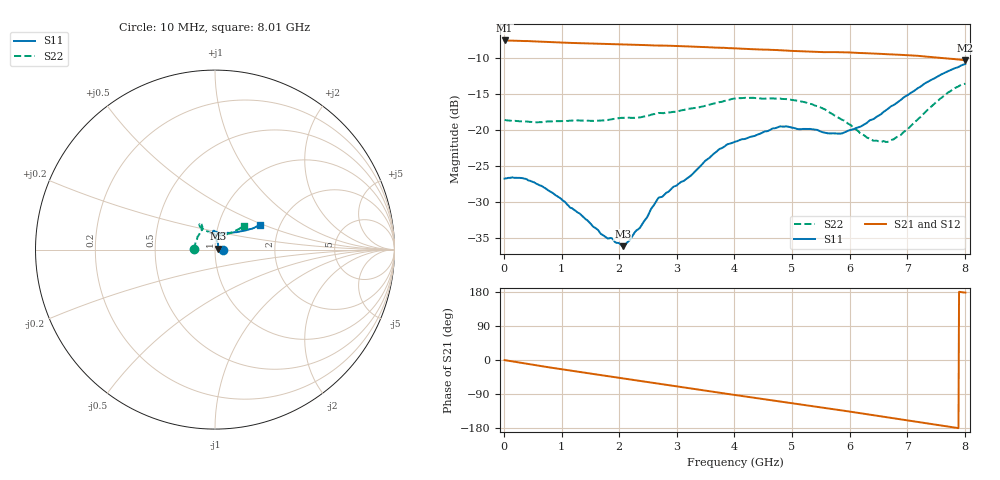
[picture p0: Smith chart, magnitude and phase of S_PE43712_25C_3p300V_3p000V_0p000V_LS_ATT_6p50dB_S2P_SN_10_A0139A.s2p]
! DEVICE ID: PE43712
! File Path: z:\PE43713\PE43713_CHAR_NOM_04292014\AMB\3p300\LS_ATT_6p50dB\PE43713_AMB_3p300V_3p000V_0p000V_LS_ATT_6p50dB_S2P_SN_10_A0139A.s2p
! Serial: 10
! Lot: A0139A
! Temp: 25C
! VDD: 3.300
! VSS: 0.000
! Control_Hi: 3.000
! Control_Lo: 0.000
! Attenuation Step: 6.50dB
! Port 1: RF1
! Port 2: RF2
! ThroughPath:1-2
! IDD: 0.0001471273
! ISS: -1.096e-007
#  Hz  S  RI  R  50
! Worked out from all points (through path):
!   801 points, 10 MHz to 8.01 GHz, reference 50 ohm
!   highest |S21| = -7.63 dB at 10 MHz (marker M1); lowest = -10.4 dB at 8.01 GHz (marker M2)
!   group delay of S21, straight-line fit = 62.5 ps
!   lowest |S11| = -36.1 dB at 2.06 GHz (marker M3), VSWR 1.03, Z = 51.5 + j0.513 ohm
!   |S11| at or under -10 dB: start of sweep to end of sweep
!   |S22| runs from -21.7 to -13.6 dB; largest |S21 - S12| = 0.0014
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1e7  0.0459 -6.25e-05  0.4156 -0.00229  0.4155 -0.00229  -0.1171 0.000707
3e8  0.0457 -0.00756  0.4088 -0.0557  0.4086 -0.0557  -0.1139 0.01
5.4e8  0.0413 -0.0114  0.3975 -0.0965  0.3976 -0.0966  -0.1113 0.0171
9.6e8  0.0314 -0.0127  0.3692 -0.1612  0.3693 -0.1612  -0.1103 0.0312
1.35e9  0.0234 -0.00989  0.3357 -0.2131  0.3357 -0.2131  -0.107 0.0439
1.71e9  0.0184 -0.00333  0.2993 -0.2557  0.2994 -0.2557  -0.1005 0.0578
2.06e9  0.0148 0.00498  0.2592 -0.2919  0.2592 -0.2918  -0.0969 0.0724
2.15e9  0.0152 0.00702  0.248 -0.3003  0.2481 -0.3002  -0.0948 0.0756
2.37e9  0.0152 0.0148  0.2195 -0.3189  0.2194 -0.3188  -0.0872 0.0854
2.68e9  0.0176 0.0287  0.1779 -0.3393  0.1779 -0.3393  -0.0777 0.1049
3.23e9  0.0104 0.0464  0.0984 -0.3641  0.0984 -0.3642  -0.0727 0.1195
3.72e9  0.00565 0.0722  0.0271 -0.3694  0.0268 -0.3694  -0.0732 0.1362
4.01e9  -0.000122 0.0826  -0.015 -0.3663  -0.015 -0.3662  -0.0802 0.1437
4.79e9  -0.00921 0.105  -0.1189 -0.3349  -0.1189 -0.3352  -0.0868 0.1397
5.35e9  0.00116 0.1007  -0.1822 -0.2959  -0.1821 -0.2957  -0.0825 0.1255
5.63e9  0.013 0.0935  -0.2103 -0.2737  -0.2102 -0.2738  -0.0674 0.1149
5.88e9  0.0265 0.091  -0.2363 -0.2504  -0.2358 -0.2505  -0.0497 0.1059
6.39e9  0.0714 0.0935  -0.2764 -0.1939  -0.2759 -0.1937  -0.0052 0.0847
6.68e9  0.1044 0.0954  -0.2935 -0.1577  -0.2932 -0.1577  0.0252 0.0791
6.99e9  0.1392 0.1011  -0.3072 -0.1174  -0.3067 -0.1174  0.0556 0.0825
7.71e9  0.2225 0.1239  -0.3107 -0.0224  -0.3105 -0.0227  0.1378 0.1179
8.01e9  0.2506 0.1378  -0.3029 0.0116  -0.3024 0.0111  0.1611 0.133
